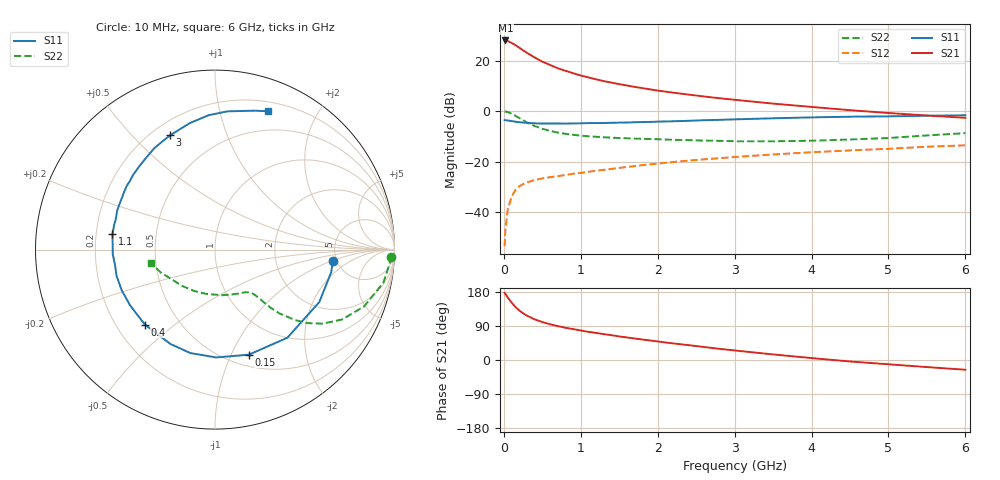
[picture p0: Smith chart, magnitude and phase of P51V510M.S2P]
! SIEMENS Small Signal Semiconductors
! BFP183
! Si NPN RF Bipolar Junction Transistor in SOT143
! VCE = 1.5 V  IC = 10 mA
! Common Emitter S-Parameters:  March  1996
# GHz  S  MA  R  50
!  f  S11  S21  S12  S22
! GHz  MAG  ANG  MAG  ANG  MAG  ANG  MAG  ANG
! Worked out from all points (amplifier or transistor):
!   36 points, 10 MHz to 6 GHz, reference 50 ohm
!   highest |S21| = 28.0 dB at 20 MHz (marker M1)
!   |S21| within 3 dB of that: start of sweep to 207.1 MHz
!   unconditionally stable (mu >= 1): 1.113 GHz to 5.722 GHz
!   at 250 MHz: K = 0.34, MSG = 26.5 dB, |S12| = -29.0 dB
!   at 1.4 GHz: K = 1.10, MAG = 15.2 dB, |S12| = -22.9 dB
!   at 6 GHz: K = 0.97, MSG = 5.5 dB, |S12| = -13.6 dB
!   S11 on the Smith chart (normalised r, x): 10 MHz: 4.66, -1.03; 150 MHz: 0.62, -1.17; 400 MHz: 0.32, -0.40; 1.1 GHz: 0.27, +0.07; 3 GHz: 0.27, +0.65; 6 GHz: 0.29, +1.42
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0.01  0.661 -5.4  24.94 177.2  0.0021 86.1  0.9828 -2.3
0.02  0.6596 -11.1  25.08 174.3  0.0044 84.9  0.9766 -4.5
0.05  0.6505 -26.7  24.46 165.1  0.0111 79.9  0.956 -11.1
0.1  0.6353 -50.6  22.44 151.8  0.0198 67.9  0.8886 -20.9
0.15  0.6152 -72.1  20.33 140.1  0.0271 59.5  0.8081 -28.8
0.2  0.6009 -89.4  18.07 130.8  0.0322 53.7  0.7283 -34.5
0.25  0.5926 -103.4  15.96 123.2  0.0355 48.7  0.6578 -38.5
0.3  0.5815 -115.3  14.28 117.1  0.0386 46.3  0.5952 -41.3
0.4  0.572 -133.1  11.54 107.3  0.0429 42.6  0.5062 -44.7
0.5  0.5659 -146.6  9.538 100.2  0.0463 40.5  0.4466 -46.3
0.6  0.5672 -156.3  8.193 94.4  0.0489 40.0  0.4045 -47.1
0.7  0.5676 -165.1  7.066 89.5  0.0513 40.0  0.3752 -47.6
0.9  0.5704 -177.5  5.629 81.6  0.0572 40.8  0.3381 -48.6
1.1  0.5776 171.4  4.638 74.3  0.0627 41.8  0.3166 -49.9
1.5  0.5891 154.8  3.419 62.2  0.0746 43.1  0.2922 -54.3
1.8  0.6065 144.2  2.848 54.1  0.0847 42.9  0.2815 -59.1
2.2  0.6276 132.1  2.318 43.8  0.0976 41.7  0.2697 -66.9
3  0.6843 111.4  1.674 25.2  0.1227 37.5  0.2524 -86.7
3.5  0.7189 101.2  1.405 14.7  0.138 34.1  0.2517 -101.1
4.5  0.7731 85.0  1.042 -3.9  0.1659 26.5  0.2732 -132.3
5.5  0.8065 73.7  0.817 -18.7  0.1964 19.6  0.3288 -157.3
6  0.8256 68.9  0.735 -25.7  0.2094 15.1  0.3647 -168.2
